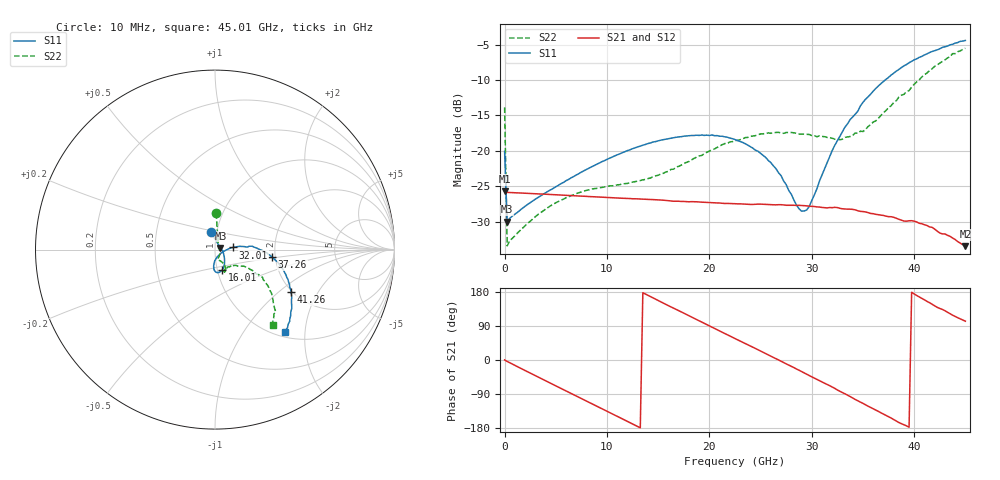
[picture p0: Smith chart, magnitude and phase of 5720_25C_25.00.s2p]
! Device:  ADRF5720
! Description: 0.5dB LSB GaAs MMIC 6-bit Digital Attenuator
! Frequency:  0.000009 -  40 GHz
! Ports:
!	RF1	= Port 1
!	RF2	= Port 2
! Vdd:  3.3 Volt
! Vss:  -3.3 Volt
! Control:  0/3.3 Volt
! State:  25.00 dB attenuation
! Data:  The device was measured using G-S-G Probes on a matrix board.
!  Data was collected using an calibrated 4 port network analyzer.
!  The reference plane for this measurement is at the launchers.
! Note:  Analog Devices supplies this data as a sample of measured data
!  for this product.  Your particular data for this product may vary.
!  Data was taken at 25 degrees C.
!  Analog Devices reserves the right to change this data at anytime.
# GHZ S DB R 45.0
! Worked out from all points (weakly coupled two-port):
!   181 points, 10 MHz to 45.01 GHz, reference 45 ohm
!   highest |S21| = -25.69 dB at 10 MHz (marker M1); lowest = -33.5 dB at 45.01 GHz (marker M2)
!   lowest |S11| = -30.0 dB at 260 MHz (marker M3), VSWR 1.07, Z = 47.8 + j0.88 ohm
!   |S11| at or under -10 dB: start of sweep to 37.17 GHz
!   |S22| runs from -33.4 to -5.5 dB; largest |S21 - S12| = 0.00021
!   S11 on the Smith chart (normalised r, x): 10 MHz: 0.94, +0.18; 16.01 GHz: 1.05, -0.25; 32.01 GHz: 1.22, +0.03; 37.26 GHz: 1.92, -0.18; 41.26 GHz: 1.97, -1.22; 45.01 GHz: 1.09, -1.57
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0.01  -20.08 103.8  -25.69 0.1  -25.67 0.1  -13.86 88.2
0.26  -30.02 16.9  -25.87 -3.8  -25.87 -3.8  -33.43 22.4
1.26  -28.70 1.4  -25.94 -17.6  -25.94 -17.6  -31.62 -8.3
4.01  -25.93 -21.9  -26.13 -54.8  -26.13 -54.8  -28.23 -47.2
7.76  -22.81 -43.2  -26.41 -105.1  -26.41 -105.1  -25.69 -71.0
15.26  -18.49 -69.2  -26.95 153.6  -26.95 153.6  -23.29 -65.8
16.01  -18.28 -71.4  -27.05 143.3  -27.05 143.3  -22.90 -64.0
20.26  -17.76 -83.7  -27.33 86.5  -27.33 86.5  -19.86 -58.7
22.76  -18.55 -91.0  -27.49 53.3  -27.49 53.3  -18.52 -60.6
26.01  -21.66 -94.0  -27.60 10.1  -27.60 10.2  -17.52 -65.3
27.01  -23.50 -91.4  -27.61 -3.3  -27.61 -3.3  -17.47 -66.4
29.01  -28.52 -54.5  -27.72 -30.5  -27.71 -30.4  -17.63 -67.7
29.51  -28.36 -36.7  -27.77 -37.7  -27.77 -37.6  -17.66 -66.3
30.26  -26.22 -11.3  -27.87 -47.8  -27.88 -47.8  -17.85 -65.7
32.01  -19.94 6.8  -28.03 -71.3  -28.03 -71.2  -18.22 -60.1
33.26  -16.62 6.9  -28.22 -89.3  -28.22 -89.3  -18.09 -51.4
35.01  -13.14 3.4  -28.58 -114.5  -28.59 -114.5  -17.27 -40.4
37.26  -9.89 -7.5  -29.23 -146.4  -29.23 -146.4  -14.29 -29.7
37.76  -9.29 -10.1  -29.31 -153.2  -29.32 -153.2  -13.62 -28.9
41.26  -6.29 -29.1  -30.55 154.7  -30.57 154.7  -9.00 -34.2
43.76  -4.94 -42.6  -32.32 118.2  -32.31 118.2  -6.26 -45.9
45.01  -4.40 -49.7  -33.47 102.4  -33.49 102.5  -5.50 -52.5
